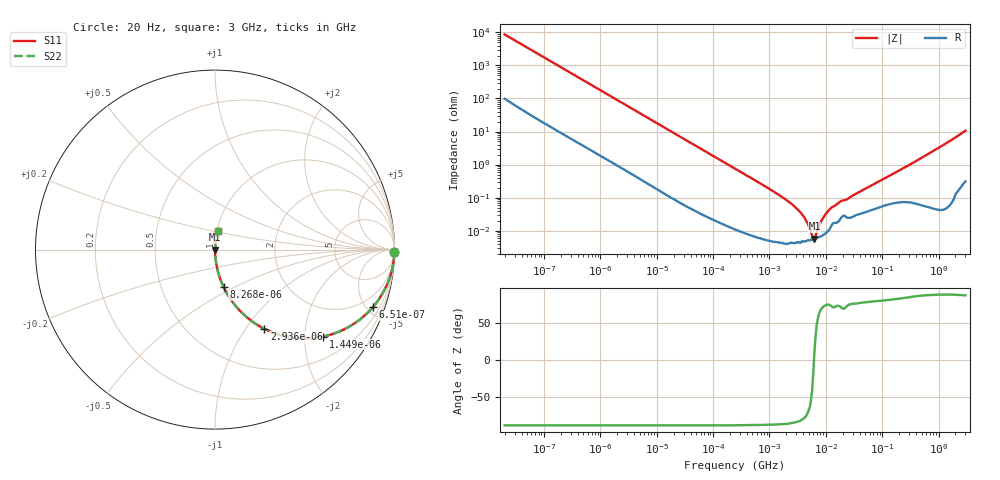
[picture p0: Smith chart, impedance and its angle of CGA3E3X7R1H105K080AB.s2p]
! S-Parameter Data Generated by TDK Corporation
! Copyright(C) 2025 TDK Corporation.
! All Rights Reserved.
! TDK P/N: CGA3E3X7R1H105K080AB (Multilayer Ceramic Chip Capacitor)
! Property: C=1uF
! Size(LxWxT): 1.6x0.8x0.8mm
! Model Type: s2p (Touchstone File Format Version 1.0)
! Frequency: DC=Yes Start=2E-05MHz Stop=3000MHz 402points Log-sweep
! Model Generated on July 30, 2025
! Terms and conditions regarding TDK Simulation Models:
! 1)This simulation model is being provided solely for informational
!  purposes. Please refer to the specifications of the products in
!  terms of detailed characteristics of such products.
! 2)In no event shall TDK Corporation of any of its subsidiaries be
!  liable for any loss or damage arising, directly or indirectly,
!  from any information contained in this simulation model, including,
!  but not limited to loss or damages arising from any inaccuracies,
!  omissions or errors in connection with such information.
! 3)Any and all copyrights on this simulation model are owned by
!  TDK Corporation.  Duplication or redistribution of this simulation
!  model without prior written permission from TDK Corporation
!  is prohibited.
! 4)This simulation model is subject to any modification or change
!  without any prior notice.
! 5)Neither TDK Corporation nor any of its subsidiaries shall make any
!  warranty, express or implied, including but not limited to the
!  correctness, implied warranties of merchantability and fitness for
!  a particular purpose with respect to this simulation models.
! 6)The use of this simulation model shall be deemed to have consented
!  to the terms and conditions hereof.
! Port Assignments:
!  1 ---| |--- 2
! Applicable Conditions:
!  Temperature = 25 degC
!  DC Bias Voltage = 0 V
!  Small Signal Operation
# Hz S MA R 50
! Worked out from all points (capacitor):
!   401 points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, 20 Hz to 3 GHz, reference 50 ohm
!   read as one part in series: C = 916 nF near 21.97 Hz
!   lowest |Z| = 5.67 mohm at 6.302 MHz (marker M1)
!   series resonance near 6.177 MHz, so ESL is about 730 pH
!   S11 on the Smith chart (normalised r, x): 20 Hz: open; 651 Hz: 1.06, -5.46; 1.449 kHz: 1.03, -2.47; 2.936 kHz: 1.01, -1.22; 8.268 kHz: 1.00, -0.44; 3 GHz: 1.01, +0.21
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20  0.9998 -0.7  0.01155 88.7  0.01155 88.7  0.9998 -0.7
131.4132  0.9965 -4.3  0.07439 85.1  0.07439 85.1  0.9965 -4.3
468.3012  0.9644 -14.8  0.2546 74.7  0.2546 74.7  0.9644 -14.8
651.0388  0.9359 -20.0  0.3428 69.4  0.3428 69.4  0.9359 -20.0
1449.075  0.7727 -38.8  0.6269 50.6  0.6269 50.6  0.7727 -38.8
2935.582  0.5192 -58.1  0.8493 31.3  0.8493 31.3  0.5192 -58.1
4699.985  0.3567 -68.5  0.9306 20.9  0.9306 20.9  0.3567 -68.5
8267.595  0.2136 -77.1  0.9748 12.3  0.9748 12.3  0.2136 -77.1
10965.3  0.1633 -80.0  0.985 9.4  0.985 9.4  0.1633 -80.0
37279.19  0.04925 -86.6  0.9983 2.8  0.9983 2.8  0.04925 -86.6
244949  0.0076 -88.7  0.9999 0.4  0.9999 0.4  0.0076 -88.7
1157719  0.001569 -88.2  1 0.1  1 0.1  0.001569 -88.2
2458367  0.0006482 -86.1  1 0.0  1 0.0  0.0006482 -86.1
3754991  0.0003186 -81.4  1 0.0  1 0.0  0.0003186 -81.4
5735495  6.928e-05 -40.6  0.9999 0.0  0.9999 0.0  6.928e-05 -40.6
6301608  5.67e-05 12.0  0.9999 -0.0  0.9999 -0.0  5.67e-05 12.0
7257249  0.0001154 57.1  0.9999 -0.0  0.9999 -0.0  0.0001154 57.1
9625281  0.0002924 74.2  0.9999 -0.0  0.9999 -0.0  0.0002924 74.2
1.2766e7  0.000507 73.0  0.9999 -0.0  0.9999 -0.0  0.000507 73.0
1.34297e8  0.004583 81.8  0.9994 -0.3  0.9994 -0.3  0.004583 81.8
9.695178e8  0.031 87.4  0.9991 -1.8  0.9991 -1.8  0.031 87.4
3e9  0.1054 82.3  0.9913 -6.0  0.9913 -6.0  0.1054 82.3
